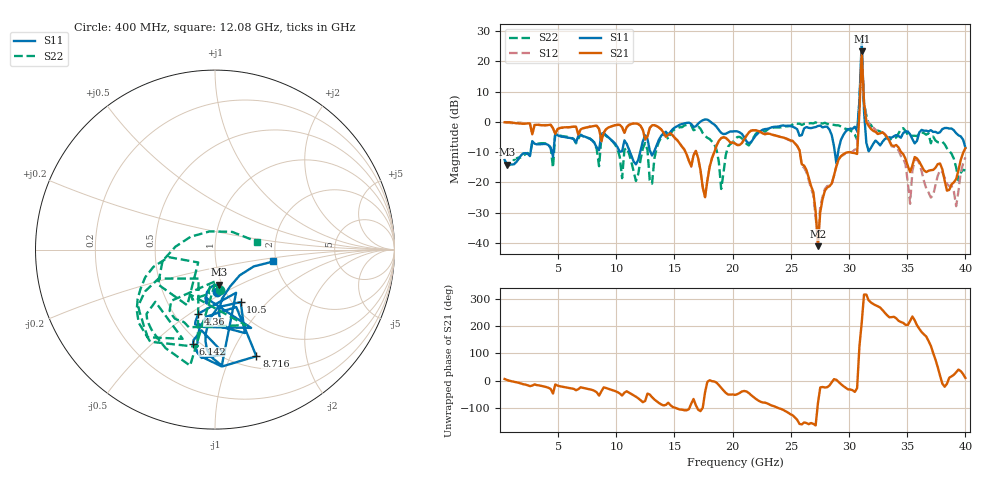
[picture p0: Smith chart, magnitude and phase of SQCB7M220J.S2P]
! Network Analyzer HP8722ES.07.66: Jul 25, 2000 Serial No. US39175408
! 27 Oct 2004  08:39:19
! Frequency  S11  S21  S12  S22
# HZ  S  DB R  50
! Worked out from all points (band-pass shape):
!   201 points, 400 MHz to 40 GHz, reference 50 ohm
!   highest |S21| = 23.30 dB at 31.09 GHz (marker M1); lowest = -41.0 dB at 27.33 GHz (marker M2)
!   |S21| within 3 dB of the highest: 31.06082 GHz to 31.12484 GHz (64.02 MHz wide, 0.206 % of centre)
!   lowest |S11| = -14.1 dB at 598 MHz (marker M3), VSWR 1.49, Z = 48.2 - j19.7 ohm
!   |S11| at or under -10 dB: start of sweep to 2.63 GHz; 4.455 GHz to 4.595 GHz (139.8 MHz wide, 3.09 % of centre); 11.18 GHz to 12.05 GHz (877.1 MHz wide, 7.55 % of centre)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
!   |S22| runs from -22.2 to 21.0 dB; largest |S21 - S12| = 0.86
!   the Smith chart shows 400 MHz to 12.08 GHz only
!   S11 on the Smith chart (normalised r, x): 400 MHz: 0.92, -0.46; 4.36 GHz: 0.65, -0.54; 6.142 GHz: 0.46, -0.68; 8.716 GHz: 0.63, -1.26; 10.5 GHz: 1.09, -0.71; 12.08 GHz: 1.94, -0.29
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4e8  -12.52 -87.0  -0.14 5.7  -0.05 7.3  -12.90 -82.7
5.98e8  -14.09 -83.8  -0.17 2.3  -0.24 3.1  -13.93 -88.6
4.36e9  -8.66 -104.6  -0.95 -31.2  -0.95 -30.5  -8.51 -130.5
6.142e9  -5.40 -103.2  -1.68 -28.4  -1.68 -28.9  -5.28 -133.9
7.132e9  -4.74 -99.8  -2.10 -26.7  -2.20 -28.0  -4.72 -133.1
8.716e9  -3.91 -68.8  -6.36 -39.8  -6.59 -38.5  -5.18 -100.1
1.0498e10  -9.75 -63.9  -1.78 -55.2  -1.87 -56.2  -18.58 -142.5
1.2082e10  -9.57 -11.5  -1.29 -72.2  -1.32 -73.7  -12.47 10.7
1.3666e10  -5.87 2.4  -1.90 -82.8  -1.85 -83.4  -6.54 -3.0
1.7626e10  0.78 -10.8  -24.85 -43.3  -24.77 -40.6  -4.62 -90.2
2.02e10  -3.11 -7.0  -7.15 -52.9  -7.14 -53.3  -5.65 -17.9
2.4358e10  -1.19 -26.0  -5.17 -108.5  -5.17 -109.7  -1.57 -16.0
2.6932e10  -1.86 -161.5  -23.16 -159.6  -24.14 -158.5  -0.52 -29.1
2.7328e10  -1.38 175.8  -41.00 -83.3  -36.88 -48.2  -0.60 -32.3
3.0694e10  -2.96 94.7  -10.59 -28.0  -8.99 -27.7  -5.86 -60.6
3.0892e10  6.74 17.4  2.94 125.5  7.09 122.3  6.87 -47.3
3.109e10  26.83 -90.2  23.30 -146.8  23.61 -147.7  21.03 152.6
3.1288e10  3.54 -47.1  6.25 -43.0  6.73 -42.5  6.24 -68.4
3.1684e10  -9.73 -66.2  -1.29 -64.0  -0.38 -65.7  -0.55 -59.7
3.3466e10  -5.08 -107.1  -6.27 -126.9  -6.45 -131.6  -6.11 -47.7
3.5248e10  -4.13 -137.2  -16.57 -140.5  -27.03 1.9  -4.79 -62.1
4e10  -8.47 -152.2  -8.67 9.6  -11.73 7.5  -16.04 84.4
